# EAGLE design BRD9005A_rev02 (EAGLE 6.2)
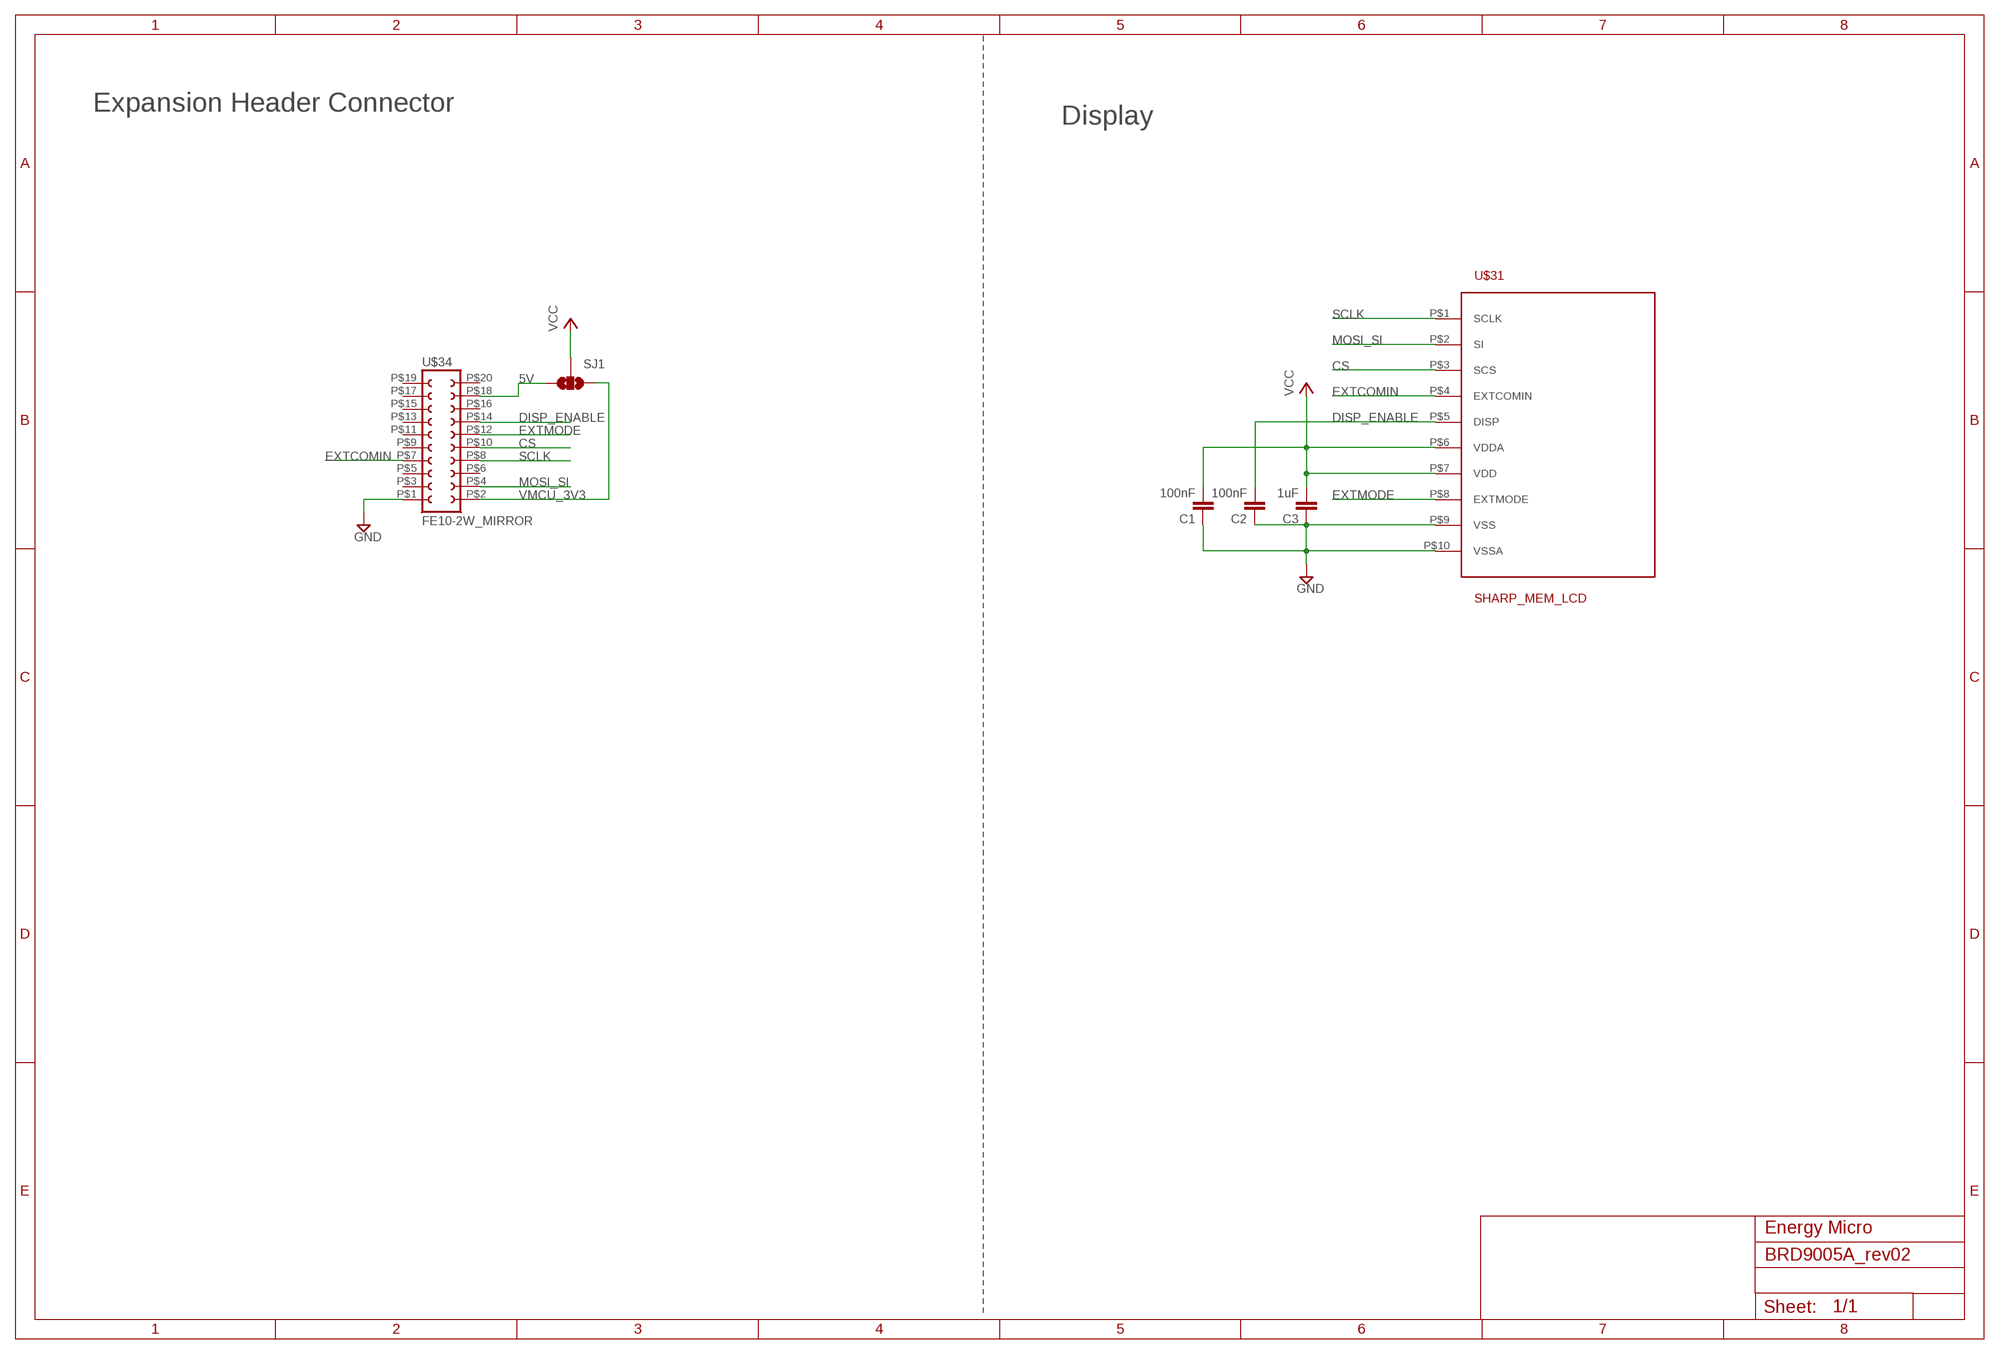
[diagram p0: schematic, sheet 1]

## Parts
C1  100nF  C-EUC0402K  [C0402K]
C2  100nF  C-EUC0402K  [C0402K]
C3  1uF  C-EUC0402K  [C0402K]
SJ1  SOLDERJUMPER_2WAYT  [SJ_2]
U$31  SHARP_MEM_LCD  [SHARP_MEM_LCD]
U$34  FE10-2W_MIRROR  [FE10-2W_MIRROR]

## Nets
5V: SJ1.3 U$34.P$18
CS: U$31.P$3(SCS) U$34.P$10
DISP_ENABLE: C2.2 U$31.P$5(DISP) U$34.P$14
EXTCOMIN: U$31.P$4(EXTCOMIN) U$34.P$7
EXTMODE: U$31.P$8(EXTMODE) U$34.P$12
GND: C1.1 C2.1 C3.1 U$31.P$9(VSS) U$31.P$10(VSSA) U$34.P$1
MOSI_SI: U$31.P$2(SI) U$34.P$4
SCLK: U$31.P$1(SCLK) U$34.P$8
VCC: C1.2 C3.2 SJ1.2 U$31.P$6(VDDA) U$31.P$7(VDD)
VMCU_3V3: SJ1.1 U$34.P$2
Unconnected: U$34.P$3 U$34.P$5 U$34.P$6 U$34.P$9 U$34.P$11 U$34.P$13 U$34.P$15 U$34.P$16 U$34.P$17 U$34.P$19 U$34.P$20

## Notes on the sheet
- Expansion Header Connector
- Display
- Energy Micro

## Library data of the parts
C1-C3 = rcl:C-EU: CAPACITOR, European symbol
SJ1 = SparkFun_mod:SOLDERJUMPER_2WAY: Solder Jumper 2 way solder jumper
U$31 = sharp_mem_lcd:SHARP_MEM_LCD
U$34 = con-lsta:FE10-2W_MIRROR

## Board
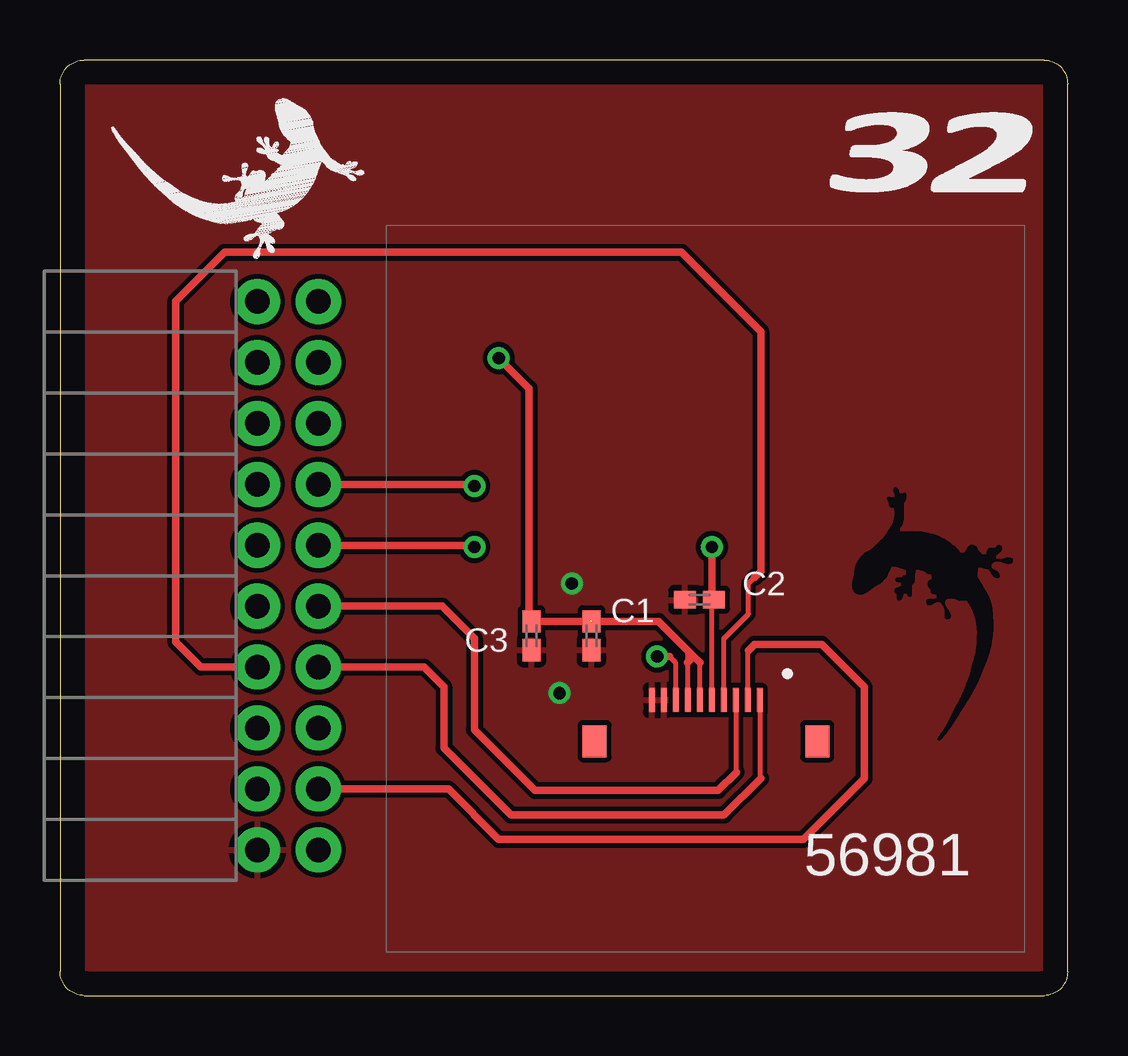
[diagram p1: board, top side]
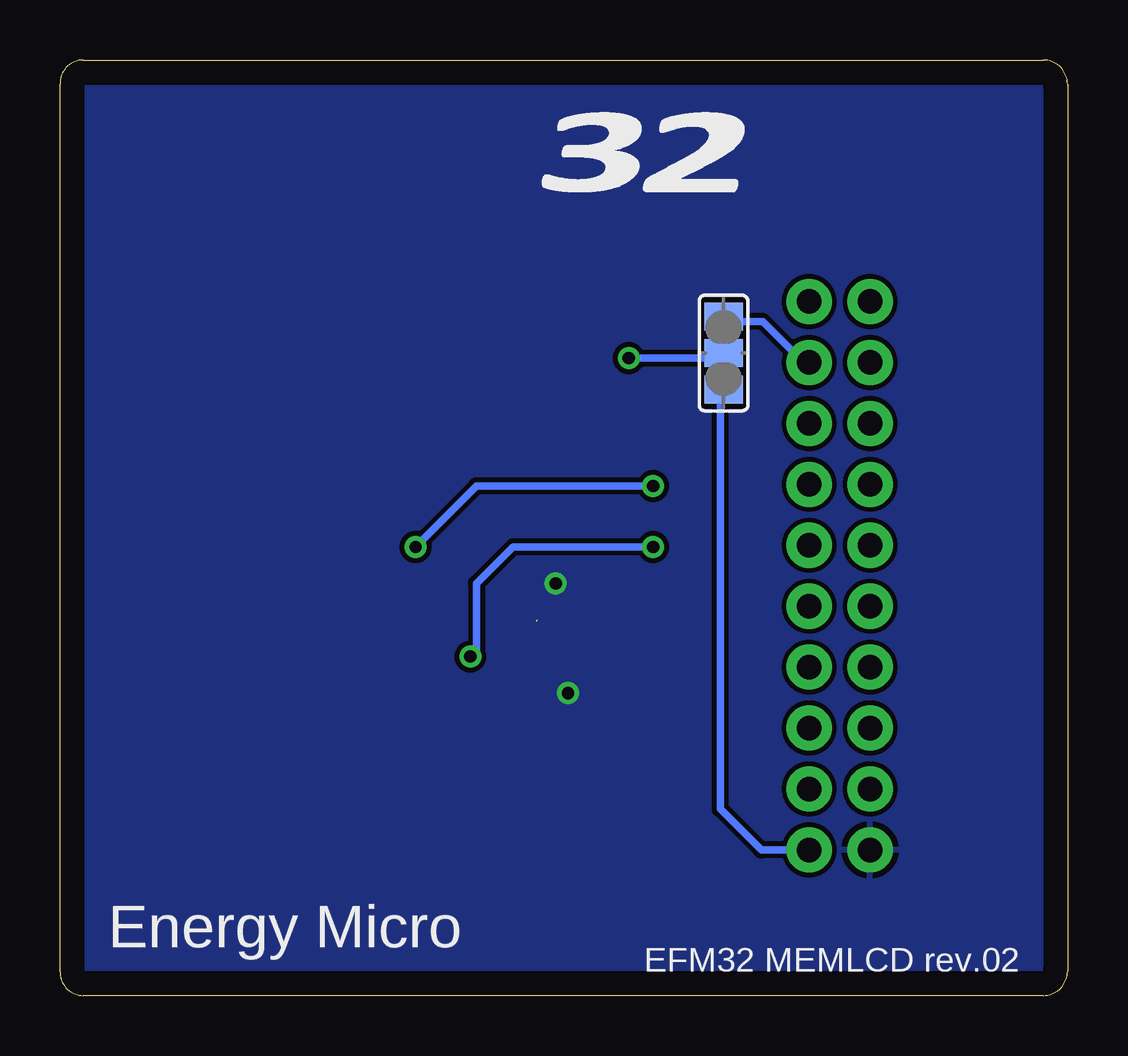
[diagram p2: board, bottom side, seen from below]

Size 42 x 39 mm. Coordinates in mm from the lower left corner, seen from the top.
Outline: 1.02,0 41.03,0 arc90 42,1 42,38 arc90 41.03,39 1.02,39 arc90 0,37.98 0,1.02 arc90 1.02,0
Copper layers (1*16): Top 0.035mm / dielectric 1.5mm / Bottom 0.035mm
Design rules: minimum track width 8mil, minimum drill 20mil, track to track 8mil, track to pad 8mil, pad to pad 8mil, via to via 8mil, smd to smd 8mil, copper to edge 40mil, drill to drill 8mil, minimum pad ring 10mil, minimum via ring 8mil, stop-mask expansion 4mil, vias tented up to drill 20mil, thermal gap 10mil

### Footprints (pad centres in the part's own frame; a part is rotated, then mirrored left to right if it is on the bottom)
C0402K = smd 0.925 x 0.74: 1 -0.6,0; 2 0.6,0
SJ_2 = smd 1.168 x 1.6: 1 -1.524,0; 2 0,0; 3 1.524,0
SHARP_MEM_LCD = smd 0.25 x 1: P$1 2.25,0; P$2 1.75,0; P$3 1.25,0; P$4 0.75,0; P$5 0.25,0; P$6 -0.25,0; P$7 -0.75,0; P$8 -1.25,0; P$9 -1.75,0; P$10 -2.25,0 | smd 1 x 1.34: P$11 -4.64,-1.72; P$12 4.64,-1.72
FE10-2W_MIRROR = drill 1.016 pad 1.88: P$1 11.43,-1.27; P$2 11.43,1.27; P$3 8.89,-1.27; P$4 8.89,1.27; P$5 6.35,-1.27; P$6 6.35,1.27; P$7 3.81,-1.27; P$8 3.81,1.27; P$9 1.27,-1.27; P$10 1.27,1.27; P$11 -1.27,-1.27; P$12 -1.27,1.27; P$13 -3.81,-1.27; P$14 -3.81,1.27; P$15 -6.35,-1.27; P$16 -6.35,1.27; P$17 -8.89,-1.27; P$18 -8.89,1.27; P$19 -11.43,-1.27; P$20 -11.43,1.27

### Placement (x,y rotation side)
C1  22.16,15 90 top
C2  26.66,16.5 0 top
C3  19.66,15 90 top
SJ1  14.34,26.78 90 bottom
U$1  [EFM32_COMBINED_BOTTOM]  27,34 0 top
U$2  [EFM32_COMBINED_TOP]  27,34 0 top
U$3  [GECKO_NEG_COPPER_TOP]  36,15 0 top
U$4  [GECKO]  6.47,35.29 250 top
U$5  [GECKO_SOLDER_MASK_BOTTOM]  7,35 270 top
U$6  [GECKO_SOLDER_MASK_TOP]  35.38,25.18 0 top
U$31  26.92,12.32 0 top
U$34  9.5,17.5 270 top

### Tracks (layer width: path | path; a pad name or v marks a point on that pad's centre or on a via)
5V
  Bottom 0.305: U$34.P$18 10.99,26.39 12.7,28.1 14.22,28.1 14.48,28.35 14.22,28.35 14.27,28.31 SJ1.3
CS
  Top 0.203: U$31.P$3 28.17,9.32 28.19,9.3
  Top 0.305: U$34.P$10 15.93,16.23 17.27,14.89 17.27,11.08 19.81,8.54 27.43,8.54 28.19,9.3
DISP_ENABLE  (via drill 0.51)
  Top 0.203: U$31.P$5 27.17,16.41 C2.2
  Top 0.305: U$34.P$14 17.2,21.31 v17.27,21.24 | v27.18,18.7 27.18,16.58 C2.2
  Bottom 0.305: v17.27,21.24 24.64,21.24 v27.18,18.7
EXTCOMIN
  Top 0.203: U$31.P$4 27.67,14.88 28.7,15.91 28.7,17.18 28.96,17.43
  Top 0.305: 28.96,17.43 29.21,17.69 29.21,27.69 25.91,30.99 6.86,30.99 4.83,28.96 4.83,14.73 5.87,13.69 U$34.P$7
EXTMODE  (via drill 0.51)
  Top 0.203: U$31.P$8 25.67,13.86 25.4,14.13
  Top 0.305: U$34.P$12 17.2,18.77 v17.27,18.7 | v24.89,14.13 25.4,14.13
  Bottom 0.305: v17.27,18.7 23.11,18.7 24.64,17.18 24.64,14.38 v24.89,14.13
GND  (via drill 0.51)
  other vias: 21.34,17.18 20.83,12.61
  pour Bottom: 0,39.12 42.16,39.12 42.16,0 0,0
  pour Top: 0,39.12 42.16,39.12 42.16,0 0,0
MOSI_SI
  Top 0.203: U$31.P$2 28.67,14.36 28.7,14.38
  Top 0.305: U$34.P$4 16.19,8.61 18.29,6.51 30.99,6.51 33.53,9.05 33.53,12.86 31.75,14.64 28.96,14.64 28.7,14.38
SCLK
  Top 0.203: U$31.P$1 29.17,9.09 29.21,9.05
  Top 0.305: U$34.P$8 15.17,13.69 16,12.86 16,10.32 18.8,7.53 27.69,7.53 29.21,9.05
VCC  (via drill 0.51)  (1 unrouted)
  Top 0.203: 26.16,14.38 26.16,13.88 26.16,12.59 U$31.P$7 | U$31.P$6 26.67,13.87 26.67,13.88
  Top 0.305: 22.1,15.65 22.04,15.6 C3.2 19.56,15.7 19.56,25.31 v18.29,26.58 | C1.2 24.95,15.6 26.16,14.38 26.42,14.13 | 26.42,14.13 26.67,13.88 | 26.42,14.13 26.16,13.88
  Bottom 0.305: v18.29,26.58 14.73,26.58 14.48,26.83 14.38,26.83 SJ1.2
VMCU_3V3
  Bottom 0.305: U$34.P$2 12.77,6.07 14.48,7.78 14.48,25.12 SJ1.1

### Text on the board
_tsilk: 56981
_bsilk: EFM32 MEMLCD rev.02 | Energy Micro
